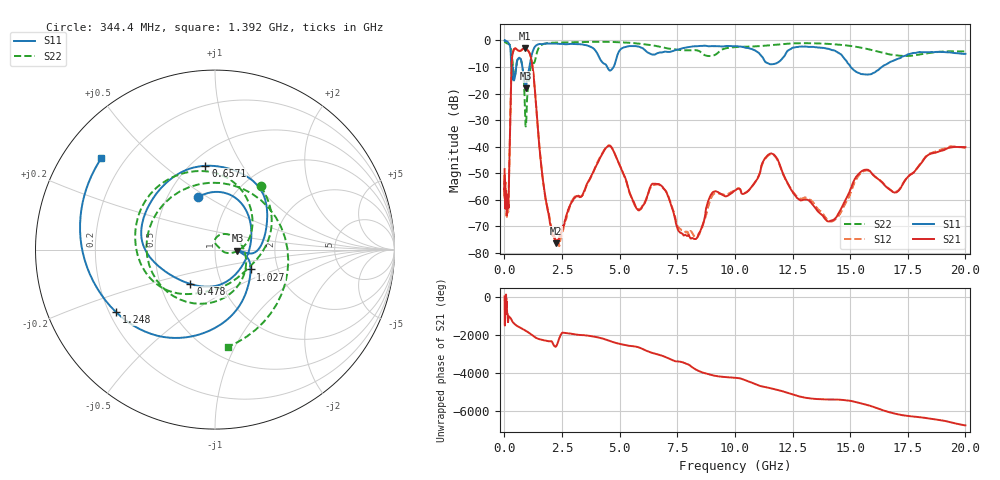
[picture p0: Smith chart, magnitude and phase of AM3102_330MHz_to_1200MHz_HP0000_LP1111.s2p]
! Date/Time: Tue, Sep 11, 2018 5:09 PM
! Network Analyzer: Agilent Technologies E8362B Rev: A.07.50.63
! Sweep from 0.010 to 20.000 GHz, 1601 Points, Sweep Type: LOG
! Power Supply: 4.950 V, 0.001 A
# Hz S DB R 50
!freq MagS11 AngS11 MagS21 AngS21 MagS12 AngS12 MagS22 AngS22
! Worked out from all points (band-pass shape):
!   1601 points, 10 MHz to 20 GHz, reference 50 ohm
!   highest |S21| = -2.98 dB at 886.4 MHz (marker M1); lowest = -76.4 dB at 2.228 GHz (marker M2)
!   |S21| within 3 dB of the highest: 339.4 MHz to 1.138 GHz (798.5 MHz wide, 108 % of centre)
!   lowest |S11| = -18.1 dB at 920.7 MHz (marker M3), VSWR 1.29, Z = 64.3 - j0.7 ohm
!   |S11| at or under -10 dB: 781.2 MHz to 1.086 GHz (305 MHz wide, 32.7 % of centre); 4.457 GHz to 4.737 GHz (279.7 MHz wide, 6.08 % of centre); 15.03 GHz to 16.37 GHz (1.347 GHz wide, 8.58 % of centre)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
!   |S22| runs from -32.4 to -0.3 dB; largest |S21 - S12| = 0.013
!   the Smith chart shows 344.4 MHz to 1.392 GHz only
!   S11 on the Smith chart (normalised r, x): 344.4 MHz: 0.70, +0.45; 478 MHz: 0.71, -0.29; 657.1 MHz: 0.59, +0.70; 1.027 GHz: 1.45, -0.34; 1.248 GHz: 0.23, -0.27; 1.392 GHz: 0.12, +0.35
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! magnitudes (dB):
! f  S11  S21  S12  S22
! 10 MHz  0.0  -48.5  -52.0  -0.3
! 35.55 MHz  0.0  -61.0  -60.6  -0.6
! 126.4 MHz  -0.4  -59.5  -63.6  -1.1
! 179.6 MHz  -0.9  -61.8  -59.2  -1.3
! 344.4 MHz  -10.3  -5.7  -5.8  -7.2
! 447.2 MHz  -14.0  -3.0  -3.1  -13.7
! 478 MHz  -12.6  -3.0  -3.0  -12.4
! 657.1 MHz  -6.6  -3.9  -4.0  -6.5
! 886.4 MHz  -16.7  -3.0  -3.0  -25.0
! 920.7 MHz  -18.1  -3.0  -3.1  -32.2
! 1.027 GHz  -12.9  -3.8  -3.8  -17.6
! 1.248 GHz  -3.7  -11.6  -11.7  -8.5
! 1.392 GHz  -1.8  -26.1  -26.5  -5.3
! 1.59 GHz  -1.4  -46.3  -46.2  -1.8
! 2.228 GHz  -1.2  -76.4  -75.6  -0.8
! 4.479 GHz  -10.3  -39.9  -39.8  -0.5
! 5.652 GHz  -2.1  -61.6  -62.0  -1.0
! 6.707 GHz  -4.6  -54.1  -54.3  -2.3
! 8.188 GHz  -2.2  -74.5  -73.1  -3.7
! 11.58 GHz  -9.0  -42.5  -42.9  -1.8
! 14.07 GHz  -3.2  -68.2  -67.8  -1.3
! 20 GHz  -5.1  -40.2  -40.5  -4.2
